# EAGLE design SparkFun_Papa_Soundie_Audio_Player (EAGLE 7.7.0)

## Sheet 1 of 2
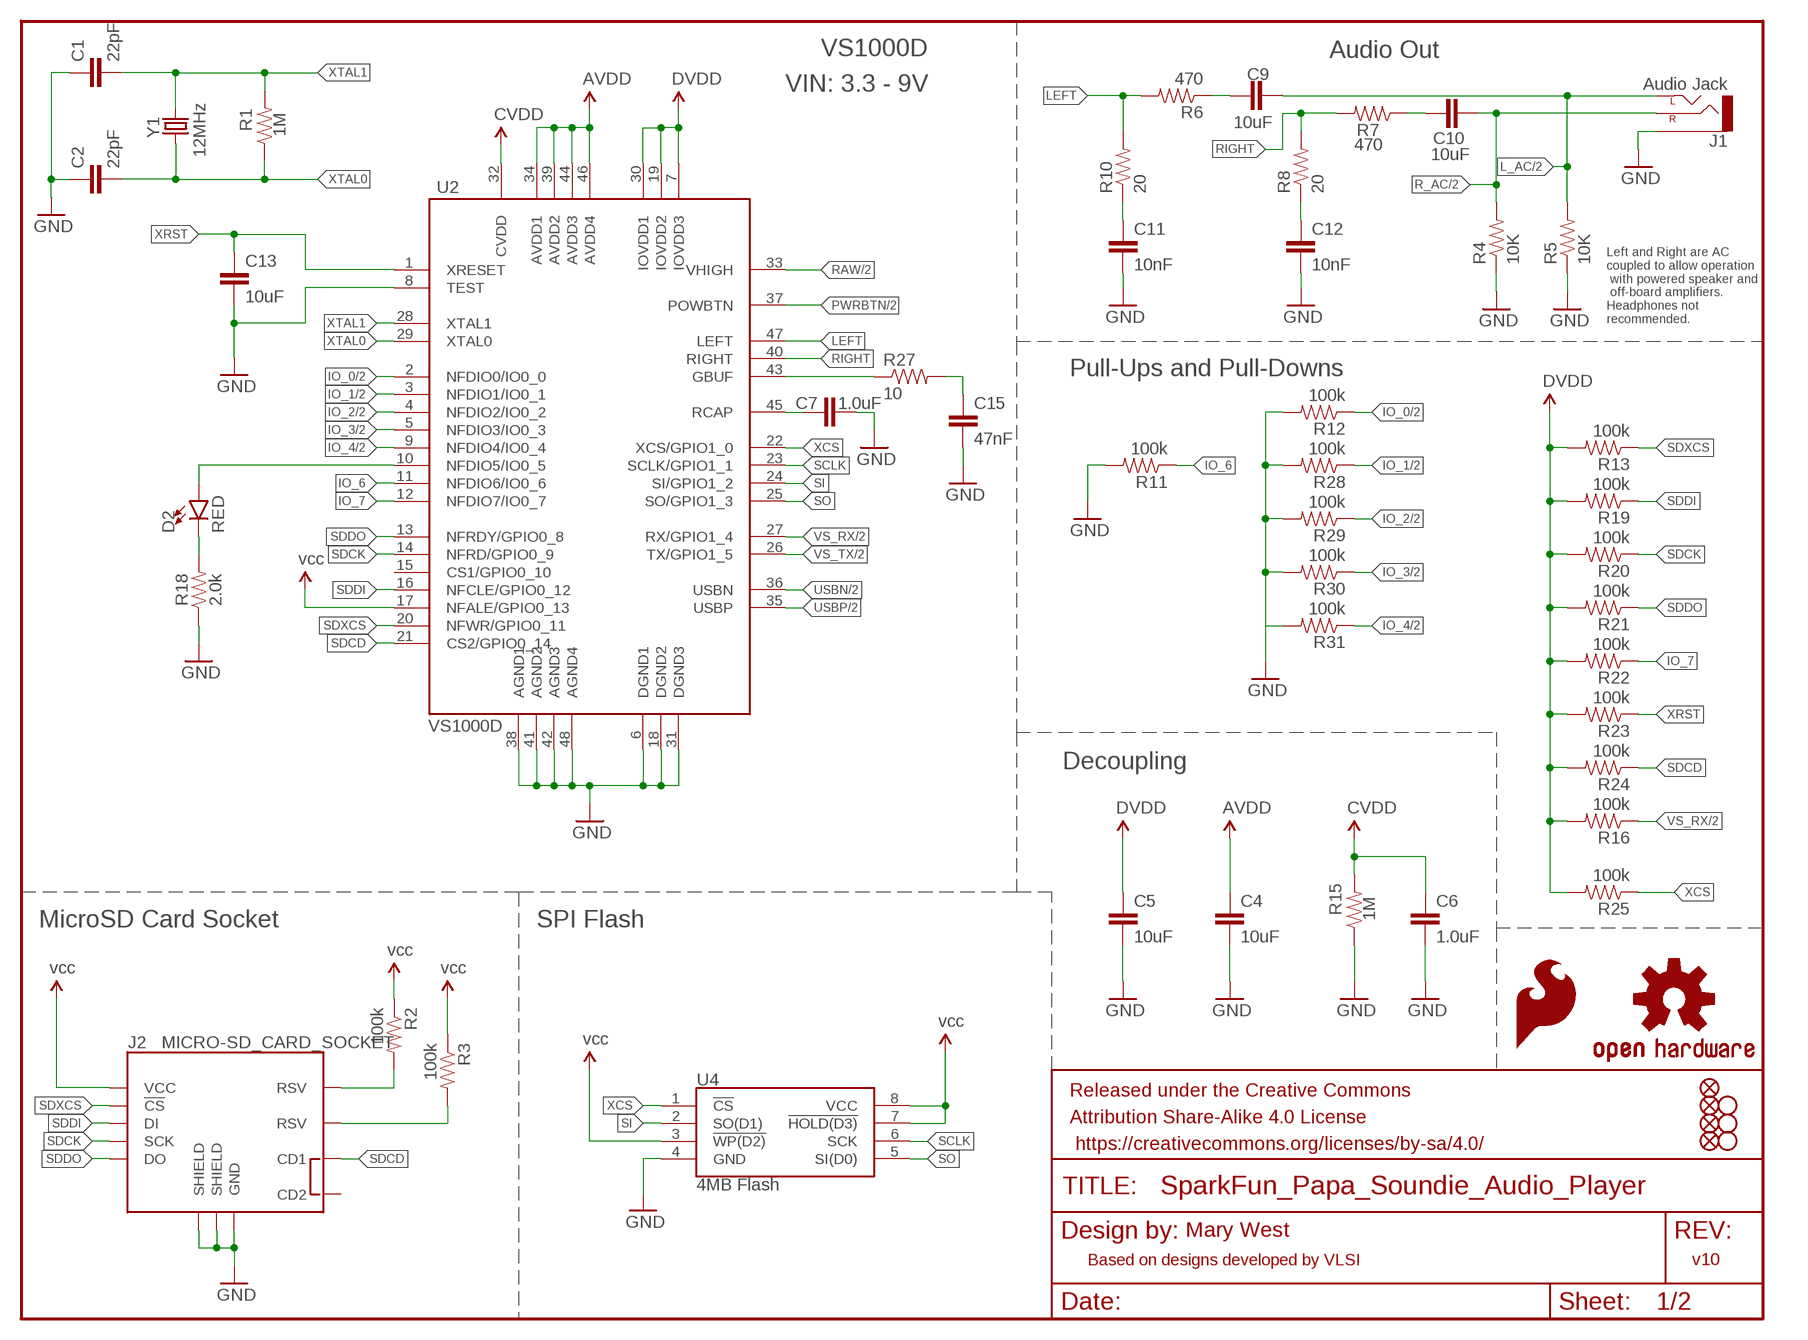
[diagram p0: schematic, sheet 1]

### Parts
C1  22pF  22PF-50V-5%(0603)  [0603-CAP]
C2  22pF  22PF-50V-5%(0603)  [0603-CAP]
C4  10uF  10UF-0603-6.3V-20%  [0603]
C5  10uF  10UF-0603-6.3V-20%  [0603]
C6  1.0uF  1.0UF-16V-10%(0603)  [0603-CAP]
C7  1.0uF  1.0UF-16V-10%(0603)  [0603-CAP]
C9  10uF  10UF-6.3V-20%(0603)  [0603-CAP]
C10  10uF  10UF-6.3V-20%(0603)  [0603-CAP]
C11  10nF  10NF/10000PF-50V-10%(0603)  [0603-CAP]
C12  10nF  10NF/10000PF-50V-10%(0603)  [0603-CAP]
C13  10uF  10UF-6.3V-20%(0603)  [0603-CAP]
C15  47nF  47NF(0.047UF/47000PF)-25V-5%(0603)SMD  [0603-CAP]
D2  RED  LED-RED0603  [LED-0603]
FD1  FIDUCIALUFIDUCIAL  [FIDUCIAL-MICRO]
FD2  FIDUCIALUFIDUCIAL  [FIDUCIAL-MICRO]
FD3  FIDUCIALUFIDUCIAL  [FIDUCIAL-MICRO]
FD4  FIDUCIALUFIDUCIAL  [FIDUCIAL-MICRO]
FRAME1  FRAME-LETTER  [CREATIVE_COMMONS]
H1  STAND-OFFTIGHT  [STAND-OFF-TIGHT]
H2  STAND-OFFTIGHT  [STAND-OFF-TIGHT]
H3  STAND-OFFTIGHT  [STAND-OFF-TIGHT]
J1  Audio Jack  AUDIO-JACKSMD2  [AUDIO-JACK-3.5MM-SMD]
J2  MICRO-SD_CARD_SOCKET  [MICRO-SD-SOCKET]
LOGO1  OSHW-LOGOL  [OSHW-LOGO-L]
LOGO2  SFE_LOGO_FLAME.2_INCH  [SFE_LOGO_FLAME_.2]
R1  1M  1MOHM-1/10W-1%(0603)  [0603-RES]
R2  100k  100KOHM-1/10W-1%(0603)  [0603-RES]
R3  100k  100KOHM-1/10W-1%(0603)  [0603-RES]
R4  10K  10KOHM-1/10W-1%(0603)0603  [0603-RES]
R5  10K  10KOHM-1/10W-1%(0603)0603  [0603-RES]
R6  470  470OHM1/10W1%(0603)  [0603-RES]
R7  470  470OHM1/10W1%(0603)  [0603-RES]
R8  20  20OHM1/10W1%(0603)SMD  [0603-RES]
R10  20  20OHM1/10W1%(0603)SMD  [0603-RES]
R11  100k  100KOHM-1/10W-1%(0603)  [0603-RES]
R12  100k  100KOHM-1/10W-1%(0603)  [0603-RES]
R13  100k  100KOHM-1/10W-1%(0603)  [0603-RES]
R15  1M  1MOHM-1/10W-1%(0603)  [0603-RES]
R16  100k  100KOHM-1/10W-1%(0603)  [0603-RES]
R18  2.0k  2.0KOHM-0603-1/10W-5%  [0603]
R19  100k  100KOHM-1/10W-1%(0603)  [0603-RES]
R20  100k  100KOHM-1/10W-1%(0603)  [0603-RES]
R21  100k  100KOHM-1/10W-1%(0603)  [0603-RES]
R22  100k  100KOHM-1/10W-1%(0603)  [0603-RES]
R23  100k  100KOHM-1/10W-1%(0603)  [0603-RES]
R24  100k  100KOHM-1/10W-1%(0603)  [0603-RES]
R25  100k  100KOHM-1/10W-1%(0603)  [0603-RES]
R27  10  10OHM-1/10W-5%0603SMD  [0603-RES]
R28  100k  100KOHM-1/10W-1%(0603)  [0603-RES]
R29  100k  100KOHM-1/10W-1%(0603)  [0603-RES]
R30  100k  100KOHM-1/10W-1%(0603)  [0603-RES]
R31  100k  100KOHM-1/10W-1%(0603)  [0603-RES]
U2  VS1000D  VS1000  [LQFP-48]
U4  4MB Flash  AT25SF041  [SO08]
Y1  12MHz  CRYSTALCRYSTAL-SMD-5X3-12MHZ  [CRYSTAL-SMD-5X3]

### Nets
AVDD: C4.1 U2.34(AVDD1) U2.39(AVDD2) U2.44(AVDD3) U2.46(AVDD4)
CVDD: C6.1 R15.2 U2.32(CVDD)
DVDD: C5.1 R13.2 R16.2 R19.2 R20.2 R21.2 R22.2 R23.2 R24.2 R25.2 U2.7(IOVDD3) U2.19(IOVDD2) U2.30(IOVDD1)
GBUF: R27.1 U2.43(GBUF)
GND: C1.1 C2.1 C4.2 C5.2 C6.2 C7.2 C11.2 C12.2 C13.2 C15.2 J1.SLEEVE J2.GND J2.GND1(SHIELD) J2.GND3(SHIELD) R4.1 R5.1 R11.2 R12.2 R15.1 R18.1 R28.2 R29.2 R30.2 R31.2 U2.6(DGND1) U2.8(TEST) U2.18(DGND2) U2.31(DGND3) U2.38(AGND1) U2.41(AGND2) U2.42(AGND3) U2.48(AGND4) U4.4(GND) ; also sheet 2
IO_0: R12.1 U2.2(NFDIO0/IO0_0) ; also sheet 2
IO_1: R28.1 U2.3(NFDIO1/IO0_1) ; also sheet 2
IO_2: R29.1 U2.4(NFDIO2/IO0_2) ; also sheet 2
IO_3: R30.1 U2.5(NFDIO3/IO0_3) ; also sheet 2
IO_4: R31.1 U2.9(NFDIO4/IO0_4) ; also sheet 2
IO_6: R11.1 U2.11(NFDIO6/IO0_6)
IO_7: R22.1 U2.12(NFDIO7/IO0_7)
L_AC: C9.2 J1.TIP(LEFT) R5.2 ; also sheet 2
LEFT: R6.2 R10.2 U2.47(LEFT)
N$2: C15.1 R27.2
N$3: C9.1 R6.1
N$6: C11.1 R10.1
N$7: C7.1 U2.45(RCAP)
N$15: J2.RSV1(RSV) R2.2
N$17: C10.1 R7.1
N$19: J2.RSV2(RSV) R3.2
N$20: C12.1 R8.1
N$34: D2.C R18.2
N$35: D2.A U2.10(NFDIO5/IO0_5)
PWRBTN: U2.37(POWBTN) ; also sheet 2
R_AC: C10.2 J1.RING(RIGHT) R4.2 ; also sheet 2
RAW: U2.33(VHIGH) ; also sheet 2
RIGHT: R7.2 R8.2 U2.40(RIGHT)
SCLK: U2.23(SCLK/GPIO1_1) U4.6(SCK)
SDCD: J2.CD1 R24.1 U2.21(CS2/GPIO0_14)
SDCK: J2.SCLK(SCK) R20.1 U2.14(NFRD/GPIO0_9)
SDDI: J2.DI R19.1 U2.16(NFCLE/GPIO0_12)
SDDO: J2.DO R21.1 U2.13(NFRDY/GPIO0_8)
SDXCS: J2.CS(!CS) R13.1 U2.20(NFWR/GPIO0_11)
SI: U2.24(SI/GPIO1_2) U4.2(SO(D1))
SO: U2.25(SO/GPIO1_3) U4.5(SI(D0))
USBN: U2.36(USBN) ; also sheet 2
USBP: U2.35(USBP) ; also sheet 2
VCC: J2.VCC R2.1 R3.1 U2.17(NFALE/GPIO0_13) U4.3(!WP(D2)) U4.7(!HOLD(D3)) U4.8(VCC) ; supply symbol labelled vcc ; also sheet 2
VS_RX: R16.1 U2.27(RX/GPIO1_4) ; also sheet 2
VS_TX: U2.26(TX/GPIO1_5) ; also sheet 2
XCS: R25.1 U2.22(XCS/GPIO1_0) U4.1(!CS)
XRST: C13.1 R23.1 U2.1(XRESET)
XTAL0: C2.2 R1.1 U2.29(XTAL0) Y1.1
XTAL1: C1.2 R1.2 U2.28(XTAL1) Y1.3
Unconnected: J2.CD2 U2.15(CS1/GPIO0_10)

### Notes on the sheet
- VS1000D | Audio Out
- VIN: 3.3 - 9V
- Left and Right are AC
  coupled to allow operation
   with powered speaker and
   off-board amplifiers.
  Headphones not 
  recommended.
- Pull-Ups and Pull-Downs
- Decoupling
- MicroSD Card Socket | SPI Flash
- Mary West
- Based on designs developed by VLSI | v10

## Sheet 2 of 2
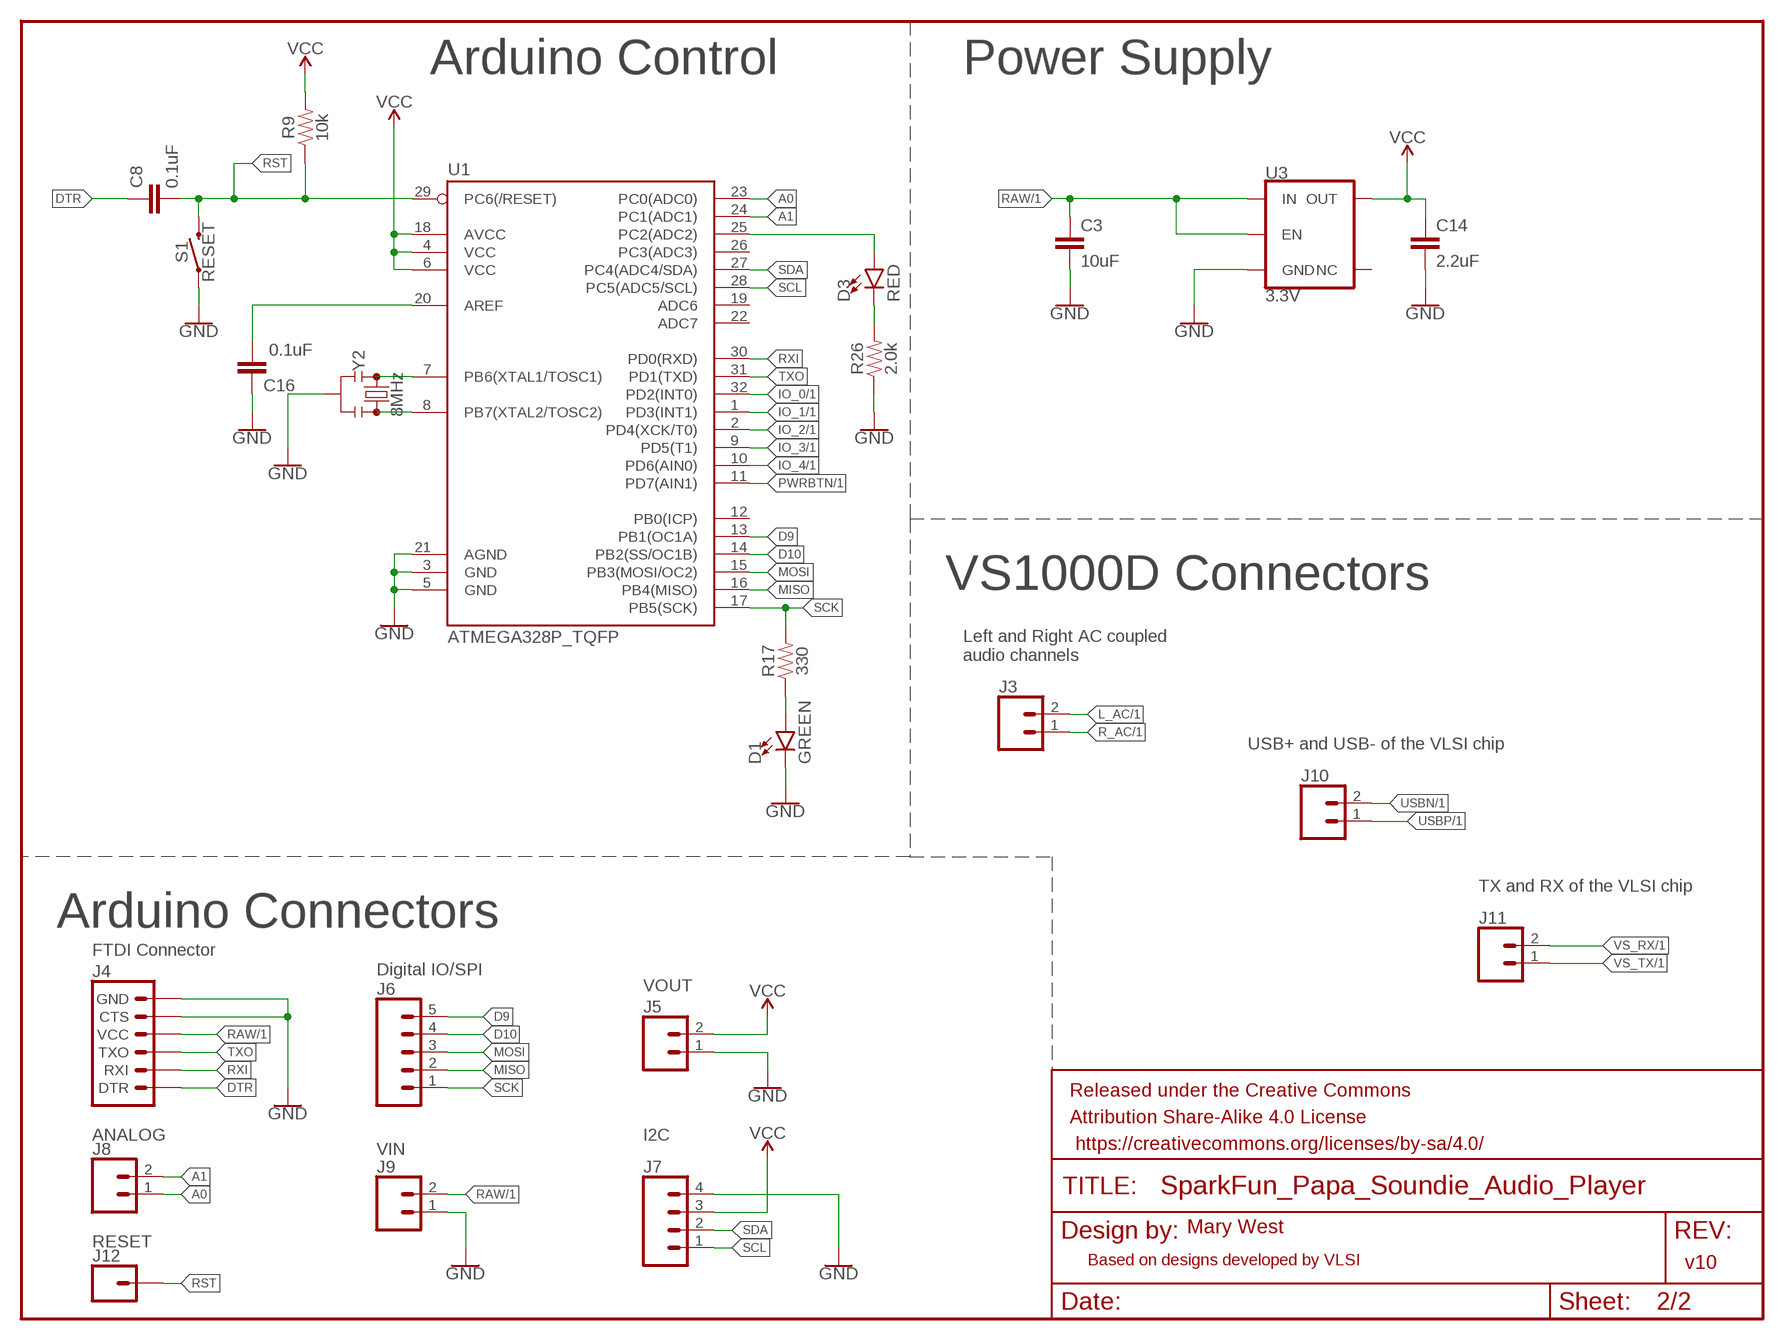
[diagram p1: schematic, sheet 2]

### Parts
C3  10uF  10UF-0603-6.3V-20%  [0603]
C8  0.1uF  0.1UF-0603-25V-(+80/-20%)  [0603]
C14  2.2uF  2.2UF-0603-10V-20%  [0603]
C16  0.1uF  0.1UF-0603-25V-(+80/-20%)  [0603]
D1  GREEN  LED-GREEN0603  [LED-0603]
D3  RED  LED-RED0603  [LED-0603]
FRAME2  FRAME-LETTER  [CREATIVE_COMMONS]
J3  CONN_02  [1X02]
J4  6_PIN_SERIAL_TARGETSILK  [6_PIN_SERIAL_TARGET_SIDE_W_SILK]
J5  CONN_02  [1X02]
J6  CONN_05  [1X05]
J7  CONN_04  [1X04]
J8  CONN_02  [1X02]
J9  CONN_02  [1X02]
J10  CONN_02  [1X02]
J11  CONN_02  [1X02]
J12  CONN_01  [1X01]
R9  10k  10KOHM-0603-1/10W-1%  [0603]
R17  330  330OHM-0603-1/10W-1%  [0603]
R26  2.0k  2.0KOHM-0603-1/10W-5%  [0603]
S1  RESET  MOMENTARY-SWITCH-SPST-SMD-5.2MM  [TACTILE_SWITCH_SMD_5.2MM]
U1  ATMEGA328P_TQFP  [TQFP32-08]
U3  3.3V  V_REG_AP2112K-3.3V  [SOT23-5]
Y2  8MHz  RESONATOR-8MHZSMD_3.2X1.3  [RESONATOR-SMD-3.2X1.3]

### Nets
A0: J8.1 U1.23(PC0(ADC0))
A1: J8.2 U1.24(PC1(ADC1))
D9: J6.5 U1.13(PB1(OC1A))
D10: J6.4 U1.14(PB2(SS/OC1B))
DTR: C8.1 J4.P$1(DTR)
GND: C3.2 C14.2 C16.1 D1.C J4.P$5(CTS) J4.P$6(GND) J5.1 J7.4 J9.1 R26.1 S1.1 U1.3(GND) U1.5(GND) U1.21(AGND) U3.2(GND) Y2.2 ; also sheet 1
IO_0: U1.32(PD2(INT0)) ; also sheet 1
IO_1: U1.1(PD3(INT1)) ; also sheet 1
IO_2: U1.2(PD4(XCK/T0)) ; also sheet 1
IO_3: U1.9(PD5(T1)) ; also sheet 1
IO_4: U1.10(PD6(AIN0)) ; also sheet 1
L_AC: J3.2 ; also sheet 1
MISO: J6.2 U1.16(PB4(MISO))
MOSI: J6.3 U1.15(PB3(MOSI/OC2))
N$8: U1.7(PB6(XTAL1/TOSC1)) Y2.1
N$16: U1.8(PB7(XTAL2/TOSC2)) Y2.3
N$31: D3.A U1.25(PC2(ADC2))
N$36: D3.C R26.2
N$39: C16.2 U1.20(AREF)
N$42: D1.A R17.1
PWRBTN: U1.11(PD7(AIN1)) ; also sheet 1
R_AC: J3.1 ; also sheet 1
RAW: C3.1 J4.P$4(VCC) J9.2 U3.1(IN) U3.3(EN) ; also sheet 1
RST: C8.2 J12.1 R9.1 S1.3 U1.29(PC6(/RESET))
RXI: J4.P$3(RXI) U1.30(PD0(RXD))
SCK: J6.1 R17.2 U1.17(PB5(SCK))
SCL: J7.1 U1.28(PC5(ADC5/SCL))
SDA: J7.2 U1.27(PC4(ADC4/SDA))
TXO: J4.P$2(TXO) U1.31(PD1(TXD))
USBN: J10.2 ; also sheet 1
USBP: J10.1 ; also sheet 1
VCC: C14.1 J5.2 J7.3 R9.2 U1.4(VCC) U1.6(VCC) U1.18(AVCC) U3.5(OUT) ; also sheet 1
VS_RX: J11.2 ; also sheet 1
VS_TX: J11.1 ; also sheet 1
Unconnected: U1.12(PB0(ICP)) U1.19(ADC6) U1.22(ADC7) U1.26(PC3(ADC3)) U3.4(NC)

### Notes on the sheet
- Arduino Control | Power Supply
- VS1000D Connectors
- Left and Right AC coupled 
  audio channels
- USB+ and USB- of the VLSI chip
- TX and RX of the VLSI chip
- Arduino Connectors
- FTDI Connector
- Digital IO/SPI
- VOUT
- ANALOG | I2C
- VIN
- Mary West
- RESET
- Based on designs developed by VLSI | v10

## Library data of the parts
C1 C2 = SparkFun-Capacitors:22PF-50V-5%(0603): CAP-07876; PROD_ID: CAP-07876
C3-C5 = SparkFun-Capacitors:10UF: 10.0µF ceramic capacitors; PROD_ID: CAP-11015
C6 C7 = SparkFun-Capacitors:1.0UF-16V-10%(0603): CAP-00868; PROD_ID: CAP-00868
C8 C16 = SparkFun-Capacitors:0.1UF: 0.1µF ceramic capacitors; PROD_ID: CAP-00810
C9 C10 C13 = SparkFun-Capacitors:10UF-6.3V-20%(0603): CAP-11015; PROD_ID: CAP-11015
C11 C12 = SparkFun-Capacitors:10NF/10000PF-50V-10%(0603): CAP-00867; PROD_ID: CAP-00867
C14 = SparkFun-Capacitors:2.2UF: 2.2µF ceramic capacitors; PROD_ID: CAP-07888
C15 = SparkFun-Capacitors:47NF(0.047UF/47000PF)-25V-5%(0603): CAP-08605; PROD_ID: CAP-08605
D1 = SparkFun-LED:LED-GREEN: Green SMD LED; PROD_ID: DIO-00821
D2 D3 = SparkFun-LED:LED-RED: Red SMD LED; PROD_ID: DIO-00819
FD1-FD4 = SparkFun-Aesthetics:FIDUCIAL: Fiducial Alignment Points
FRAME1 FRAME2 = SparkFun-Aesthetics:FRAME-LETTER: Schematic Frame - Letter
H1-H3 = SparkFun-Electromechanical:STAND-OFF: #4 Stand Off
J1 = SparkFun-Connectors:AUDIO-JACK: 3.5mm Audio Jack Simple 3.5mm common PCB mount audio jack. Variant PTH is our storefront SKU PRT-08032; PROD_ID: CONN-10353
J2 = SparkFun-Connectors:MICRO-SD_CARD_SOCKET: microSD Socket for Transflash Push-push type µSD socket. tDoc lines correctly indicate media card edge positions when inserting (unlocked, locked, depressed). NOTE: CD1 and CD2 are connected internally, and the default detect state of the socket is detect pin to ground. SparkFun Products: WAV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; PROD_ID: CONN-07820; SF_ID: PRT-00127
J3 J5 J8-J11 = SparkFun-Connectors:CONN_02: Multi connection point. Often used as Generic Header-pin footprint for 0.1 inch spaced/style header connections
J4 = SparkFun-Connectors:6_PIN_SERIAL_TARGET: 6-pin header connection for use with the "FTDI BASIC" pinout - TARGET SIDE. Also known as "Arduino Serial Program Header". It is used to mate with our FTDI Basic serial programmers using the Arduino IDE. Note, this device has "TARGET" in the name. It is intended to be used on a design that contains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
J6 = SparkFun-Connectors:CONN_05: Multi connection point. Often used as Generic Header-pin footprint for 0.1 inch spaced/style header connections On any of the 0.1 inch spaced packages, you can populate with these: Break Away Headers - Straight (PRT-00116) Break Away Male Headers - Right Angle (PRT-00553) Female Headers (PRT-00115)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
J7 = SparkFun-Connectors:CONN_04: Multi connection point. Often used as Generic Header-pin footprint for 0.1 inch spaced/style header connections On any of the 0.1 inch spaced packages, you can populate with these: Break Away Headers - Straight (PRT-00116) Break Away Male Headers - Right Angle (PRT-00553) Female Headers (PRT-00115)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; PROD_ID: CONN-09696
J12 = SparkFun-Connectors:CONN_01: Single connection point. Often used as Generic Header-pin footprint for 0.1 inch spaced/style header connections
LOGO1 = SparkFun-Aesthetics:OSHW-LOGO: Open-Source Hardware (OSHW) Logo
LOGO2 = SparkFun-Aesthetics:SFE_LOGO_FLAME: SparkFun Flame Logo
R1 R15 = SparkFun-Resistors:1MOHM-1/10W-1%(0603): RES-07868; PROD_ID: RES-07868
R2 R3 R11-R13 R16 R19-R25 R28-R31 = SparkFun-Resistors:100KOHM-1/10W-1%(0603): RES-07828; PROD_ID: RES-07828
R4 R5 = SparkFun-Resistors:10KOHM-1/10W-1%(0603): RES-00824; PROD_ID: RES-00824
R6 R7 = SparkFun-Resistors:470OHM1/10W1%(0603): RES-07869; PROD_ID: RES-07869
R8 R10 = SparkFun-Resistors:20OHM1/10W1%(0603): RES-07862; PROD_ID: RES-07862
R9 = SparkFun-Resistors:10KOHM: 10kΩ resistor; PROD_ID: RES-00824
R17 = SparkFun-Resistors:330OHM: 330Ω resistor; PROD_ID: RES-00818
R18 R26 = SparkFun-Resistors:2.0KOHM: 2kΩ resistor; PROD_ID: RES-08296
R27 = SparkFun-Resistors:10OHM-1/10W-5%0603: RES-09834; PROD_ID: RES-09834
S1 = SparkFun-Switches:MOMENTARY-SWITCH-SPST: Momentary Switch (Pushbutton) - SPST; PROD_ID: SWCH-08247; SF_SKU: COM-08720
U1 = SparkFun-IC-Microcontroller:ATMEGA328P_TQFP: Popular 328P in QFP Storefront component: ATmega328 - TQFP (COM-13448) Datasheet SparkFun Products SparkFun RedBoard - Programmed with Arduino (DEV-12757) Arduino Pro Mini 328 - 5V/16MHz (DEV-11113) Arduino Pro Mini 328 - 3.3V/8MHz (DEV-11114) SparkFun OpenLog (DEV-13712) SparkFun MicroView - OLED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; PROD_ID: IC-09069
U2 = SparkFun-IC-Conversion:VS1000: VS1000D Ogg Vorbis Player IC with USB and NAND FLASH Interface 12 MHz LQFP-48 Datasheet SparkFun Products Storefront component: Ogg Vorbis Codec IC - VS1000D (COM-08300); PROD_ID: LPA-12743
U3 = SparkFun-IC-Power:V_REG_AP2112: AP2112 - 600mA CMOS LDO Regulator w/ Enable The AP2112 is CMOS process low dropout linear regulator with enable function, the regulator delivers a guaranteed 600mA (min.) continuous load current. Features Output Voltage Accuracy: ±1.5% Output Current: 600mA (Min.) Foldback Short Current Protection: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; PROD_ID: VREG-12457
U4 = SparkFun-IC-Memory:AT25SF041: AT25SF041 4Mb Serial Flash Memory 104MHz, SPI, 8-SOIC Datasheet SparkFun Products: SparkFun ESP8266 Thing SparkFun ESP8266 Thing - Dev Board; PROD_ID: IC-12455
Y1 = SparkFun-FreqCtrl:CRYSTAL: Various standard crystals. Proven footprints.; PROD_ID: XTAL-08297
Y2 = SparkFun-Clocks:RESONATOR-8MHZ: 8MHz Resonator Digikey Example Frequency: 8MHz Frequency Stability: &plusmn;0.2% Frequency Tolerance: &plusmn;0.5% Capacitance: 33pF SparkFun Products Arduino Pro Mini 328- 3.3V/8MHz SparkFun Digital Sandbox; PROD_ID: XTAL-08895

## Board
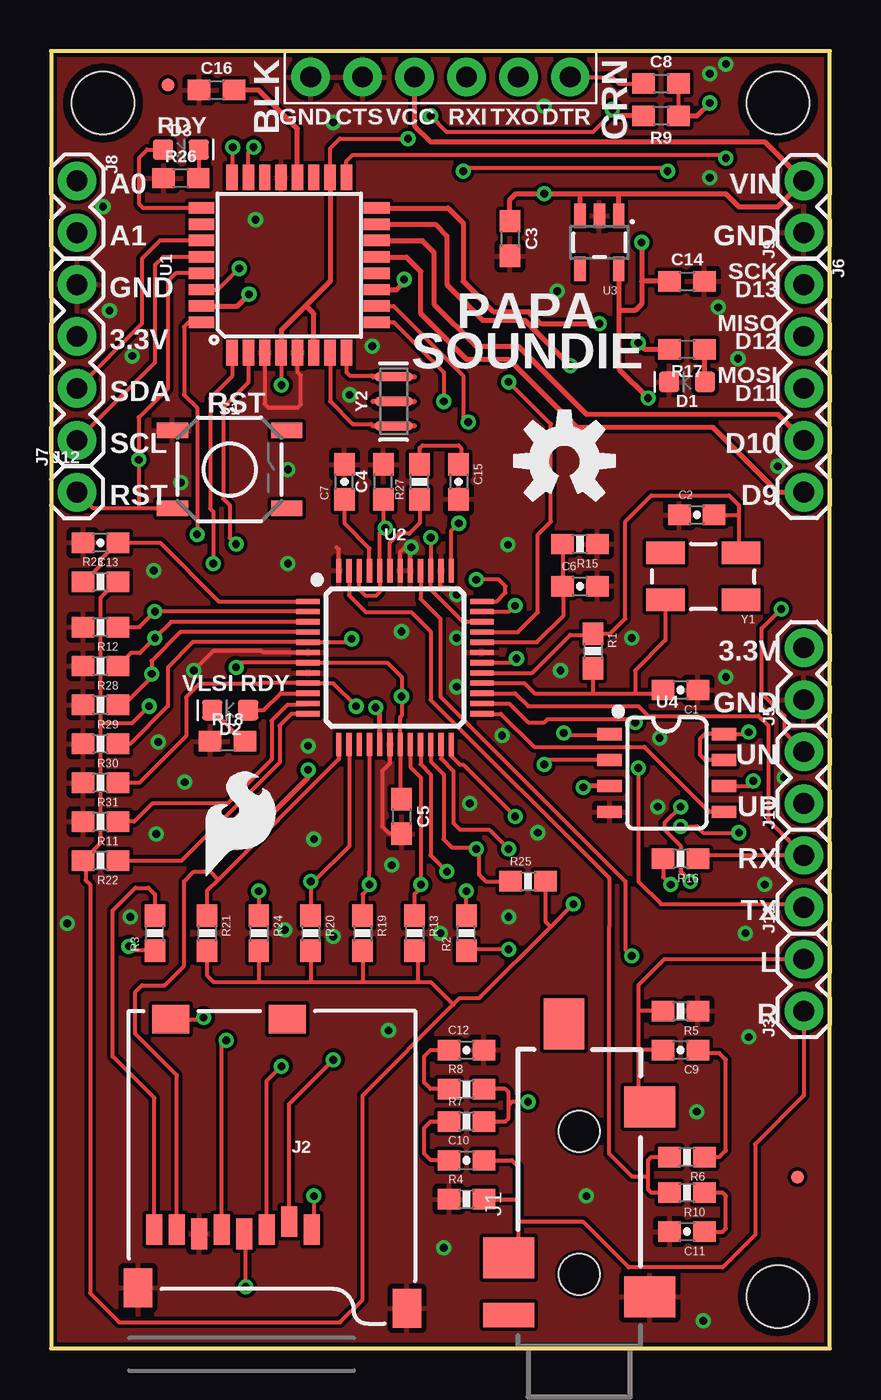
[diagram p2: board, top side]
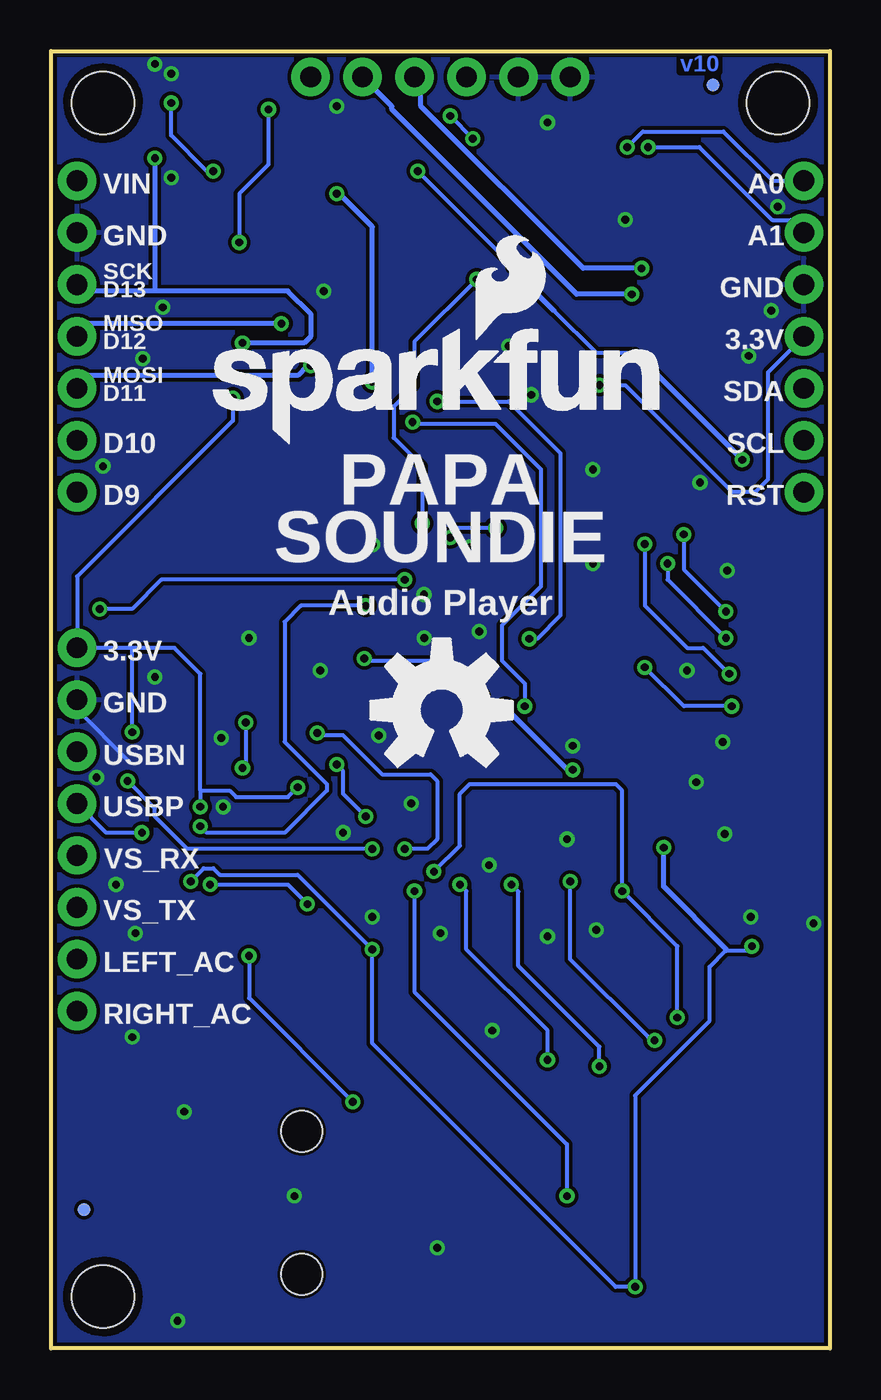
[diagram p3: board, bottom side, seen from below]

Size 38.1 x 63.5 mm. Coordinates in mm from the lower left corner, seen from the top.
Outline: 38.1,63.5 0,63.5 0,0 38.1,0 38.1,63.5
Copper layers (1*16): Top 0.035mm / dielectric 1.5mm / Bottom 0.035mm
Design rules "SparkFun-2-layer-TIGHT": minimum track width 7mil, minimum drill 15mil, track to track 7mil, track to pad 7mil, pad to pad 7mil, via to via 7mil, smd to smd 7mil, copper to edge 7mil, drill to drill 7mil, minimum pad ring 7mil, minimum via ring 7mil, stop-mask expansion 4mil, vias tented up to drill 25mil, thermal gap 10mil

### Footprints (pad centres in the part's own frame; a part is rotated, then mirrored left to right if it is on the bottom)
0603-CAP = smd 1.1 x 1: 1 -0.85,0; 2 0.85,0
0603 = smd 1.1 x 1: 1 -0.85,0; 2 0.85,0
LED-0603 = smd 1 x 1: A -0.877,0; C 0.877,0
FIDUCIAL-MICRO = smd 0.635 x 0.635: 1 0,0
STAND-OFF-TIGHT = hole 3.048: 0,0
AUDIO-JACK-3.5MM-SMD = smd 2 x 2.5: RING 4.3,3.45; SLEEVE 2.4,-3.45; TIP 11.7,-3.45 | smd 1.2 x 2.5: RSH 1.5,3.45 | smd 2.5 x 2: TSH 15.75,0.75 | hole 2: 3.5,0; 10.5,0
MICRO-SD-SOCKET = smd 1.8 x 1.4: CD1 -2.05,0.4; CD2 -7.75,0.4 | smd 0.8 x 1.5: CS -7.84,10.3; DI -6.74,10.7; DO -2.34,10.7; GND -3.44,10.9; RSV1 -8.94,10.7; RSV2 -1.24,10.7; SCLK -4.54,10.7; VCC -5.64,10.9 | smd 1.4 x 1.9: GND1 -13.6,14.55; GND3 -0.45,13.55
1X02 = drill 1.016 pad 1.88: 1 0,0; 2 2.54,0
6_PIN_SERIAL_TARGET_SIDE_W_SILK = drill 1.016 pad 1.88: P$1 -6.35,0; P$2 -3.81,0; P$3 -1.27,0; P$4 1.27,0; P$5 3.81,0; P$6 6.35,0
1X05 = drill 1.016 pad 1.88: 1 0,0; 2 2.54,0; 3 5.08,0; 4 7.62,0; 5 10.16,0
1X04 = drill 1.016 pad 1.88: 1 0,0; 2 2.54,0; 3 5.08,0; 4 7.62,0
1X01 = drill 1.016 pad 1.88: 1 0,0
0603-RES = smd 1.1 x 1: 1 -0.85,0; 2 0.85,0
TACTILE_SWITCH_SMD_5.2MM = smd 1.524 x 0.762: 1 -2.794,1.905; 2 2.794,1.905; 3 -2.794,-1.905; 4 2.794,-1.905
TQFP32-08 = smd 1.27 x 0.559: 1 -4.293,2.8; 2 -4.293,2; 3 -4.293,1.2; 4 -4.293,0.4; 5 -4.293,-0.4; 6 -4.293,-1.2; 7 -4.293,-2; 8 -4.293,-2.8; 17 4.293,-2.8; 18 4.293,-2; 19 4.293,-1.2; 20 4.293,-0.4; 21 4.293,0.4; 22 4.293,1.2; 23 4.293,2; 24 4.293,2.8 | smd 0.559 x 1.27: 9 -2.8,-4.293; 10 -2,-4.293; 11 -1.2,-4.293; 12 -0.4,-4.293; 13 0.4,-4.293; 14 1.2,-4.293; 15 2,-4.293; 16 2.8,-4.293; 25 2.8,4.293; 26 2,4.293; 27 1.2,4.293; 28 0.4,4.293; 29 -0.4,4.293; 30 -1.2,4.293; 31 -2,4.293; 32 -2.8,4.293
LQFP-48 = smd 0.254 x 1.143: 1 -2.75,-4.25; 2 -2.25,-4.25; 3 -1.75,-4.25; 4 -1.25,-4.25; 5 -0.75,-4.25; 6 -0.25,-4.25; 7 0.25,-4.25; 8 0.75,-4.25; 9 1.25,-4.25; 10 1.75,-4.25; 11 2.25,-4.25; 12 2.75,-4.25; 25 2.75,4.25; 26 2.25,4.25; 27 1.75,4.25; 28 1.25,4.25; 29 0.75,4.25; 30 0.25,4.25; 31 -0.25,4.25; 32 -0.75,4.25; 33 -1.25,4.25; 34 -1.75,4.25; 35 -2.25,4.25; 36 -2.75,4.25 | smd 1.143 x 0.254: 13 4.25,-2.75; 14 4.25,-2.25; 15 4.25,-1.75; 16 4.25,-1.25; 17 4.25,-0.75; 18 4.25,-0.25; 19 4.25,0.25; 20 4.25,0.75; 21 4.25,1.25; 22 4.25,1.75; 23 4.25,2.25; 24 4.25,2.75; 37 -4.25,2.75; 38 -4.25,2.25; 39 -4.25,1.75; 40 -4.25,1.25; 41 -4.25,0.75; 42 -4.25,0.25; 43 -4.25,-0.25; 44 -4.25,-0.75; 45 -4.25,-1.25; 46 -4.25,-1.75; 47 -4.25,-2.25; 48 -4.25,-2.75
SOT23-5 = smd 0.55 x 1.2: 1 -0.95,-1.3; 2 0,-1.3; 3 0.95,-1.3; 4 0.95,1.3; 5 -0.95,1.3
SO08 = smd 0.6 x 1.2: 1 -1.905,-2.8; 2 -0.635,-2.8; 3 0.635,-2.8; 4 1.905,-2.8; 5 1.905,2.8; 6 0.635,2.8; 7 -0.635,2.8; 8 -1.905,2.8
CRYSTAL-SMD-5X3 = smd 1.9 x 1.1: 1 -1.85,-1.15; 2 1.85,-1.15; 3 1.85,1.15; 4 -1.85,1.15
RESONATOR-SMD-3.2X1.3 = smd 0.45 x 1.905: 1 -1.2,0; 2 0,0; 3 1.2,0

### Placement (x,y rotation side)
C1  30.8,32.23 180 top
C2  31.59,40.8 0 top
C3  22.45,54.32 270 top
C4  16.26,42.42 90 top
C5  17.14,26.04 270 top
C6  25.88,37.31 0 top
C7  14.35,42.42 90 top
C8  29.84,61.91 0 top
C9  30.8,14.61 180 top
C10  20.32,9.21 0 top
C11  31.11,5.71 180 top
C12  20.32,14.61 0 top
C13  2.41,39.43 180 top
C14  31.11,52.23 0 top
C15  19.94,42.42 270 top
C16  8.1,61.59 0 top
D1  31.11,47.31 180 top
D2  8.76,31.24 180 top
D3  6.35,58.67 0 top
FD1  5.71,61.85 90 top
FD2  36.51,8.38 90 top
FD3  5.71,61.85 180 bottom
FD4  36.48,6.79 180 bottom
FRAME1  not placed on the board
FRAME2  not placed on the board
FRAME3  FRAME-LETTER  [CREATIVE_COMMONS]  not placed on the board
H1  35.56,60.96 90 top
H2  2.54,60.96 180 top
H3  35.56,2.54 0 top
J1  25.84,0.13 90 top
J2  3.81,16.51 180 top
J3  36.83,16.51 90 top
J4  19.05,62.23 180 top
J5  36.83,31.75 90 top
J6  36.83,52.07 270 top
J7  1.27,44.45 90 top
J8  1.27,57.15 270 top
J9  36.83,54.61 90 top
J10  36.83,26.67 90 top
J11  36.83,21.59 90 top
J12  1.27,41.91 0 top
LOGO1  18.99,31.24 0 bottom
LOGO2  7.24,22.86 0 top
LOGO3  OSHW-LOGOL  [OSHW-LOGO-M]  25.11,43.43 0 top
LOGO6  SFE_LOGO_NAME_FLAME.1_INCH  [SFE_LOGO_NAME_FLAME_.2]  30.87,44.2 0 bottom
R1  26.51,34.13 270 top
R2  20.32,20.32 90 top
R3  5.08,20.32 90 top
R4  20.32,7.3 0 top
R5  30.8,16.51 180 top
R6  31.11,9.37 180 top
R7  20.32,11.11 0 top
R8  20.32,12.7 0 top
R9  29.84,60.33 180 top
R10  31.11,7.62 180 top
R11  2.41,25.78 180 top
R12  2.41,35.31 180 top
R13  17.78,20.32 270 top
R15  25.88,39.37 180 top
R16  30.8,23.97 180 top
R17  31.11,48.9 180 top
R18  8.64,29.72 0 top
R19  15.24,20.32 270 top
R20  12.7,20.32 270 top
R21  7.62,20.32 270 top
R22  2.41,23.88 180 top
R23  2.41,37.53 0 top
R24  10.16,20.32 270 top
R25  23.34,22.86 0 top
R26  6.35,57.28 0 top
R27  18.03,42.42 90 top
R28  2.41,33.4 180 top
R29  2.41,31.5 180 top
R30  2.41,29.59 180 top
R31  2.41,27.69 180 top
S1  8.73,43.02 0 top
U1  11.65,53.02 90 top
U2  16.83,33.81 270 top
U3  26.83,54.13 180 top
U4  30.13,28.16 270 top
Y1  31.91,37.78 180 top
Y2  16.76,46.35 90 top

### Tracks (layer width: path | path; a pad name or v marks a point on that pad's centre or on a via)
A0  (via drill 0.38)
  Top 0.203: U1.23 9.65,58.55 v9.91,58.8 10.03,58.93
  Bottom 0.203: v9.91,58.8 9.14,59.56 5.21,59.56 2.79,57.15 J8.1
A1  (via drill 0.38)
  Top 0.203: U1.24 8.89,57.35 v8.89,58.8
  Bottom 0.203: J8.2 1.89,55.23 2.81,55.23 6.38,58.8 v8.89,58.8
AVDD  (via drill 0.38)
  Top 0.203: U2.34 20.16,35.56 18.57,37.15 U2.39 v18.57,39.69 | U2.46 15.08,37.15 15.4,36.83 15.88,36.83 16.08,37.03 U2.44 16.08,39.89 v16.35,40.16 | 16.29,40.23 v16.35,40.16 | C4.1 16.26,40.26 v16.35,40.16
  Bottom 0.203: v16.35,40.16 18.26,40.16 18.57,39.85 v18.57,39.69
CVDD
  Top 0.203: U2.32 23.77,34.56 25.08,35.88 25.08,37.25 C6.1 R15.2
D9
  Top 0.254: U1.13 17.38,53.42 18.1,52.7 18.1,50.64 20.32,48.42 22.38,48.42 25.72,45.09 32.38,45.09 35.56,41.91 J6.5
D10
  Top 0.254: U1.14 18.17,54.22 18.73,53.66 18.73,51.12 20.8,49.05 22.86,49.05 26.19,45.72 35.56,45.72 J6.4
DTR
  Top 0.203: J4.P$1 27.46,62.23 27.78,61.91 C8.1
DVDD  (via drill 0.38)
  Top 0.203: C5.1 17.08,26.95 U2.19 17.08,30.89 17.14,30.96 v17.14,31.91 17.14,32.86 16.44,33.56 U2.7 9.28,33.56 v9.05,33.34 | R21.2 7.62,18.26 7.94,17.94 10.16,17.94 | 10.16,17.94 12.7,17.94 | 12.7,17.94 15.24,17.94 | 15.24,17.94 17.94,17.94 | 17.94,17.94 18.57,17.94 19.68,16.83 | R13.2 17.94,19.31 17.94,17.94 | R19.2 15.24,17.94 | R24.2 10.16,17.94 | R20.2 12.7,17.94 | R23.2 3.21,37.53 2.41,36.73 2.41,30.61 | 2.41,30.61 2.41,24.73 R22.2 1.69,23.75 1.69,22.92 1.91,22.7 1.91,2.7 3.33,1.27 14.13,1.27 15.24,2.38 15.24,12.38 19.68,16.83 | 19.68,16.83 20,17.14 20.95,17.14 24.45,20.64 | 24.45,20.64 v25.56,21.75 | R16.2 29.95,23.07 v30.32,22.7 | U2.30 22.56,33.56 v22.77,33.77 | R25.2 24.19,20.9 24.45,20.64 | 2.41,30.61 3.97,30.61 v4.79,31.43
  Bottom 0.203: v17.14,31.91 18.89,33.66 22.65,33.66 v22.77,33.77 | v30.32,22.7 26.51,22.7 v25.56,21.75 | v4.79,31.43 7.14,31.43 v9.05,33.34
GBUF
  Top 0.203: U2.43 16.58,39.44 17.02,39.88 17.53,39.88 18.03,40.39 R27.1
GND  (via drill 0.38)
  Top 0.203: U2.6 10.39,34.06 10.32,34.13 7.94,34.13 v6.99,33.18 | U2.18 16.58,28.64 16.19,28.26 16.19,25.56 16.51,25.24 17.09,25.24 C5.2 | U1.3 10.45,46.22 10.64,46.04 12.06,46.04 12.22,46.2 12.22,47.62 12.06,47.78 12.06,48.72 U1.5 | U2.48 14.08,39.1 13.97,39.21 | U2.41 17.58,39.1 17.46,39.21 17.3,39.21 17.08,38.98 U2.42 | v19.85,36.9 19.54,37.21 19.05,37.21 19.05,38.04 U2.38
  Bottom 0.203: J5.1 36.83,31.27 34.29,28.73
  other vias: 24.92,33.18 6.35,42.39 11.59,43.02 11.59,38.42 24.13,60.8 32.23,62.39 33.02,62.87 2.54,55.88 3.97,48.58 5.02,38.07 24.77,51.75 32.64,50.96 33.61,48.45 5.24,29.69 12.86,24.92 31.59,11.59 33.97,20.32 29.69,26.51 11.43,20.48 13.81,20.16 17.62,39.21 19.84,34.77 19.84,32.38 17.14,35.08 6.54,27.72 33.02,32.86 29.77,29.89 20.48,26.67 23.81,25.24 22.38,21.11 34.92,22.7 32.23,57.31 16.67,23.65 35.88,27.94 22.07,30 16.51,15.56 19.21,4.92 26.19,7.46 34.13,15.24 31.91,1.36 14.61,46.67 15.72,49.05 10,55.24 13.81,60.01 2.86,50.8 28.42,34.77 22.35,39.34 0.79,20.8 19.05,20.32 35.56,43.18 5.14,25.18 12.57,29.5 3.87,21.11
  pour Bottom: 38.1,0 0,0 0,63.5 38.1,63.5
  pour Top: 38.1,0 0,0 0,63.5 38.1,63.5
IO_0  (via drill 0.38)
  Top 0.203: U2.2 v5.08,36.06 4.32,35.31 R12.1 | U1.32 6.72,50.22 6.51,50.01 6.51,46.67 7.14,46.04 v7.14,39.85
  Bottom 0.203: v7.14,39.85 7.14,38.13 v5.08,36.06
IO_1  (via drill 0.38)
  Top 0.203: U2.3 5.88,35.56 v5.08,34.77 4.35,34.04 3.9,34.04 R28.1 | U1.1 8.85,47.59 7.78,46.51 7.78,41.12 7.94,40.96 v7.94,38.42
  Bottom 0.203: v7.94,38.42 7.94,37.62 v5.08,34.77
IO_2  (via drill 0.38)
  Top 0.203: U2.4 6.33,35.06 4.92,33.66 v4.92,33.02 4.92,32.86 3.56,31.5 R29.1 | U1.2 9.65,47.28 8.41,46.04 8.41,41.59 8.73,41.27 8.73,39.69 v9.05,39.37
  Bottom 0.203: v9.05,39.37 9.05,36.35 6.99,34.29 6.19,34.29 v4.92,33.02
IO_3  (via drill 0.38)
  Top 0.203: U1.9 16.77,50.22 19.21,47.78 v19.21,46.35 | R30.1 3.87,29.59 5.71,31.43 5.71,33.34 6.94,34.56 U2.5 14.53,34.56 v14.7,34.73
  Bottom 0.203: v19.21,46.35 15.72,46.35 13.18,43.81 13.18,35.88 14.32,34.73 v14.7,34.73
IO_4  (via drill 0.38)
  Top 0.203: U1.10 16.76,51.02 20.16,47.62 20.16,45.59 v20.41,45.34 | v14.92,31.43 13.79,32.56 U2.9 10.21,32.56 10.16,32.51 7.24,32.51 6.6,31.88 6.6,29.97 4.32,27.69 R31.1 3.39,27.81
  Bottom 0.203: v14.92,31.43 14.92,32.54 16.03,33.66 16.03,35.4 14.13,37.31 14.13,43.02 16.35,45.24 20.32,45.24 v20.41,45.34
IO_6
  Top 0.203: U2.11 12.51,31.5 11.56,31.5 10.79,30.73 10.79,28.83 8.64,26.67 4.95,26.67 4.06,25.78 R11.1
IO_7
  Top 0.203: U2.12 11.76,31.06 11.18,30.48 11.18,28.67 7.32,24.81 7.27,24.77 6.38,23.88 R22.1
L_AC
  Top 0.203: 28.73,14.61 28.73,12.39 J1.TIP | C9.2 28.73,14.61 | J3.2 30,19.05 28.73,17.78 28.73,16.51 | 28.73,16.51 28.73,14.61 | R5.2 28.73,16.51
LEFT
  Top 0.203: R10.2 29.37,7.62 29.21,7.78 29.21,8.41 | 29.21,8.41 29.21,9.21 29.37,9.37 R6.2 | U2.47 14.58,36.86 15.4,36.04 17.62,36.04 18.57,35.08 18.57,31.75 27.3,23.02 27.3,20.64 27.3,20.16 27.3,9.53 28.42,8.41 29.21,8.41
MISO  (via drill 0.38)
  Top 0.254: U1.16 19.43,55.82 20.16,55.09 20.16,52.23 21.63,50.76 23.36,50.76 23.95,50.16 v26.83,50.16
  Bottom 0.254: v26.83,50.16 36.2,50.16 J6.2
MOSI  (via drill 0.38)
  Top 0.254: U1.15 18.8,55.02 19.37,54.45 19.37,52.07 21.11,50.32 23.18,50.32 v25.4,48.1
  Bottom 0.254: v25.4,48.1 25.56,48.1 26.04,47.62 36.2,47.62 J6.3
N$2
  Top 0.203: R27.2 18.03,44.07 18.16,44.2 19.94,44.2 20.07,44.07 20.07,43.4 C15.1
N$3
  Top 0.203: R6.1 32.7,9.37 33.02,9.68 33.02,14.13 32.7,14.45 31.81,14.45 C9.1
N$6
  Top 0.203: C11.1 32.86,5.71 33.02,5.87 33.02,7.46 32.86,7.62 R10.1
N$7
  Top 0.203: U2.45 15.58,39.16 14.35,40.39 C7.1
N$8
  Top 0.203: U1.7 13.65,46.35 14.76,45.24 15.66,45.24 15.75,45.16
N$15  (via drill 0.38)
  Top 0.203: R2.2 v20.32,22.38 | v12.86,7.46 12.86,5.92 J2.RSV1
  Bottom 0.203: v20.32,22.38 20.32,17.46 12.86,10 v12.86,7.46
N$16
  Top 0.203: U1.8 14.45,47.78 14.61,47.62 15.68,47.62 15.75,47.55
N$17
  Top 0.203: C10.1 18.57,9.21 18.26,9.53 18.26,10.79 18.57,11.11 R7.1
N$19
  Top 0.203: J2.RSV2 5.05,12.25 3.02,14.29 3.02,21.43 4.13,22.54 4.76,22.54 5.08,22.23 R3.2
N$20
  Top 0.203: R8.1 18.57,12.7 18.26,13.02 18.26,14.29 18.57,14.61 C12.1
N$31
  Top 0.203: U1.25 4.5,55.82 4.32,56.01 4.32,58.29 4.7,58.67 D3.A
N$34
  Top 0.203: D2.C 9.41,29.72 R18.2
N$35
  Top 0.203: U2.10 11.24,32.06 10.41,31.24 D2.A
N$36
  Top 0.203: D3.C 7.24,57.28 R26.2
N$39
  Top 0.254: U1.20 12.05,59.7 10.16,61.59 C16.2
N$42
  Top 0.254: R17.1 31.96,47.33 D1.A
PWRBTN  (via drill 0.38)
  Top 0.203: 19.58,38.63 U2.37 19.58,40.02 v19.94,40.39
  Top 0.254: U1.11 16.9,51.82 17.27,52.2 v17.27,52.32
  Bottom 0.203: v17.27,52.32 20.32,49.28 20.32,47.12 21.34,46.1 21.34,44.58 19.94,43.18 v19.94,40.39
R_AC
  Top 0.203: C10.2 22.54,9.21 22.86,8.89 22.86,7.3 | 22.86,7.3 22.86,6.19 | 22.86,6.19 22.86,4.89 J1.RING | R4.2 22.86,7.3 | J3.1 36.83,12.38 34.45,10 34.45,5.56 32.86,3.97 28.26,3.97 26.04,6.19 22.86,6.19
RAW  (via drill 0.38)
  Top 0.203: U2.33 22.84,35.06 23.81,36.04 23.81,39.85 24.45,40.48 24.45,45.24 v22.38,47.31
  Top 0.254: J4.P$4 17.78,59.85 18.57,59.05 34.92,59.05 J9.2 35.56,55.88 33.66,55.88 33.02,56.52 27.81,56.52 | U3.1 27.78,56.48 27.81,56.52 | 25.91,56.52 27.81,56.52 | U3.3 25.88,56.49 25.91,56.52 | C3.1 22.45,56.23 22.73,56.52 v24.13,56.52 25.91,56.52
  Bottom 0.254: v22.38,47.31 22.38,54.9 24,56.52 v24.13,56.52
RIGHT  (via drill 0.38)
  Top 0.203: R7.2 22.23,11.11 22.38,11.27 22.38,11.91 | 22.38,11.91 22.38,12.54 22.23,12.7 R8.2 | U2.40 18.08,36.69 19.05,35.72 19.05,31.91 28.1,22.86 28.1,19.53 v28.42,19.21 | v23.34,12.06 22.54,12.06 22.38,11.91
  Bottom 0.203: v28.42,19.21 28.42,17.14 v23.34,12.06
RST  (via drill 0.38)
  Top 0.203: U1.29 6.11,52.62 5.71,52.23 5.71,46.99 4.29,45.56 v4.29,43.5 4.29,41.15 4.32,41.12 | C8.2 R9.1 | v20.16,57.63 20.32,57.78 30,57.78 v30.16,57.63 | 4.32,41.12 2.06,41.12 J12.1 | S1.3 4.32,41.12
  Top 0.254: R9.1 31.59,60.33 v32.23,60.96
  Bottom 0.203: 15.56,52.86 15.56,53.02 v20.16,57.63 | v30.16,57.63 30.48,57.63 32.23,59.37 v32.23,60.96 | 13.49,50.8 11.43,48.74 9.53,48.74 8.89,48.1
  Bottom 0.254: 15.56,52.86 13.49,50.8 | 8.89,48.1 v4.29,43.5
RXI  (via drill 0.38)
  Top 0.203: U1.30 8.17,51.82 v9.21,52.86
  Bottom 0.254: v9.21,52.86 12.06,52.86 20,60.8 20,61.91 J4.P$3
SCK  (via drill 0.38)
  Top 0.203: U1.17 14.45,58.11 14.76,58.42 32.86,58.42 v33.02,58.26
  Top 0.254: R17.2 29.05,48.9 v28.73,49.21
  Bottom 0.254: 33.02,51.75 26.51,51.75 25.4,50.64 25.4,49.53 25.72,49.21 v28.73,49.21 | 33.02,51.75 36.51,51.75 J6.1 | v33.02,58.26 33.02,51.75
SCL
  Top 0.203: U1.28 5.48,53.42 5.08,53.02 5.08,48.26 J7.1
SCLK  (via drill 0.38)
  Top 0.203: U2.23 19.08,28.86 19.68,28.26 19.68,25.72 20,25.4 21.43,25.4 v22.38,24.45 | U4.6 34.11,27.53 v34.36,27.77
  Bottom 0.203: v22.38,24.45 31.43,24.45 33.02,26.04 33.02,26.43 v34.36,27.77
SDA
  Top 0.203: U1.27 5.33,54.22 4.45,53.34 4.45,50.16 J7.2
SDCD  (via drill 0.38)
  Top 0.203: U2.21 18.08,28.59 18.57,28.1 18.57,24.13 v19.37,23.34 | v10.16,22.38 R24.1 | J2.CD1 7.38,16.11 v7.46,16.19
  Bottom 0.203: v7.46,16.19 7.46,19.68 v10.16,22.38 10.16,27.3 10.48,27.62 17.62,27.62 18.1,27.15 18.1,24.61 v19.37,23.34
SDCK  (via drill 0.38)
  Top 0.203: U2.14 14.58,24.58 12.86,22.86 v12.7,22.86 R20.1 | J2.SCLK 8.35,14.86 v8.57,15.08
  Bottom 0.203: v8.57,15.08 8.57,15.24 8.89,15.24 12.7,19.05 v12.7,22.86
SDDI  (via drill 0.38)
  Top 0.203: U2.16 15.58,23.34 v15.58,22.7 15.58,22.56 15.24,22.23 R19.1 | J2.DI 10.55,13.09 v11.27,13.81
  Bottom 0.203: v11.27,13.81 11.27,14.76 15.24,18.73 15.24,22.36 v15.58,22.7
SDDO
  Top 0.203: U2.13 14.08,28.84 8.18,22.94 | 8.18,22.94 7.62,22.38 R21.1 | J2.DO 6.15,13.38 4.13,15.4 4.13,17.46 4.45,17.78 5.56,17.78 6.51,18.73 6.51,22.86 6.99,23.34 7.78,23.34 8.18,22.94
SDXCS  (via drill 0.38)
  Top 0.203: U2.20 17.58,28.46 18.1,27.94 v18.1,22.7 18.1,22.54 17.78,22.23 R13.1 | J2.CS 11.65,11.97 v13.81,14.13
  Bottom 0.203: v13.81,14.13 13.81,15.56 17.78,19.53 17.78,22.38 v18.1,22.7
SI  (via drill 0.38)
  Top 0.203: U2.24 19.58,29 20,28.57 20.16,28.57 v22.7,26.04 | U4.2 24.35,28.8 v24.13,28.57
  Bottom 0.203: 22.86,26.19 v22.7,26.04 23.81,27.15 23.81,28.26 v24.13,28.57
SO
  Top 0.203: U2.25 22.01,31.06 23.63,29.44 29.03,29.44 32.16,26.31 32.16,26.26 U4.5
TXO  (via drill 0.38)
  Top 0.254: U1.31 9.11,51.02 v9.68,51.59
  Bottom 0.254: v9.68,51.59 12.38,51.59 21.43,60.64 21.43,60.8 J4.P$2
USBN  (via drill 0.38)
  Top 0.203: U2.36 21.8,36.56 22.23,36.99 22.23,37.31 21.91,37.62 v20.8,37.62 | J10.2 35.88,30.16 35.88,30.96 34.77,32.07 34.77,35.24 v35.72,36.2
  Bottom 0.203: v20.8,37.62 32.7,37.62 34.13,36.2 v35.72,36.2
USBP  (via drill 0.38)
  Top 0.203: U2.35 22.41,36.06 v22.7,36.35 | v30.8,25.56 31.59,25.56 31.91,25.24 v33.66,25.24
  Bottom 0.203: v22.7,36.35 25.88,36.35 26.67,35.56 26.67,29.69 24.61,27.62 24.61,27.3 26.67,25.24 30.48,25.24 v30.8,25.56 | v33.66,25.24 35.4,25.24 J10.1
VCC  (via drill 0.38)
  Top 0.203: R3.1 4.03,19.47 v3.81,19.68 | v9.53,3.02 9.53,5.54 J2.VCC | 11.27,49.85 v11.27,47.15 | 29.05,46.67 v29.21,46.51 | v18.57,60.33 19.37,59.53 26.51,59.53 27.46,60.48 v27.46,60.64 | v17.46,59.21 14.13,59.21 13.65,58.74 U1.18 | v22.38,19.53 20.32,19.53 R2.1 | v31.27,22.86 30.8,23.34 30.8,24.61 30,25.4 30,25.72 v30.8,26.51 | 26.1,27.53 v26.04,27.46 | U4.7 32,28.8 31.75,29.05 31.75,29.84 31.97,30.07 U4.8 34.04,30.07 v34.13,30.16
  Top 0.254: U1.18 13.65,52.23 12.46,51.04 | 12.46,51.04 11.27,49.85 11.27,48.75 U1.4 | U1.6 12.85,50.65 12.46,51.04 | R9.2 27.78,60.33 v27.46,60.64 | U3.5 27.78,50.8 | v29.21,46.51 27.78,47.95 27.78,50.8 | v28.89,54.13 28.89,52.23 | C14.1 28.89,52.23 | 28.89,52.23 28.89,51.12 28.57,50.8 27.78,50.8 | 15.88,31.5 v15.88,31.37 16.08,31.17 U2.17 | v12.57,28.32 12.57,27.94 9.14,24.51 v8.13,24.51 | U4.3 26.04,27.53 v26.04,27.46
  Bottom 0.203: v11.27,47.15 10,47.15 4.76,41.91 3.65,41.91 3.02,42.55 3.02,47.78 J7.3 | v29.21,46.51 29.21,45.4 36.83,37.78 J5.2 34.09,34.29 | v27.46,60.64 27.46,57.94 28.89,56.52 v28.89,54.13 | v3.81,19.68 4.03,19.47 R3.1 5.87,18.68 5.87,16.03 9.53,12.38 v9.53,3.02 10.48,3.02 22.38,14.92 v22.38,19.53 26.04,23.18 29.84,23.18 30.16,23.5 30.64,23.5 v31.27,22.86 | 30.8,27.3 v30.8,26.51 | 30.8,27.3 29.37,27.3 29.05,26.99 26.51,26.99 v26.04,27.46 | v18.57,60.33 v17.46,59.21 | 30.8,27.3 30.8,33.02 32.07,34.29 34.09,34.29 | v34.13,30.16 34.13,34.25 34.09,34.29
  Bottom 0.254: v15.88,31.37 12.83,28.32 v12.57,28.32 | v8.13,24.51 8.13,22.61 5.08,19.56 R3.1
VS_RX
  Top 0.203: U2.27 22.7,32.06 23.34,31.43 28.73,31.43 29.21,30.96 34.61,30.96 35.08,30.48 35.08,25.88 J11.2 31.81,24.13 R16.1 31.43,24.19
VS_TX  (via drill 0.38)
  Top 0.203: U2.26 22.41,31.56 23.34,30.64 24.13,30.64 24.29,30.8 28.42,30.8 v28.57,30.64 | v28.73,28.42 28.73,22.86 29.84,21.75 36.67,21.75 J11.1
  Bottom 0.203: v28.57,30.64 28.57,28.57 v28.73,28.42
XCS  (via drill 0.38)
  Top 0.203: U2.22 18.58,28.73 19.21,28.1 19.21,24.92 19.61,24.53 20.72,24.53 v20.8,24.45 20.95,24.29 20.95,23.18 21.27,22.86 R25.1 | U4.1 27.27,30 25.2,30 v25.08,30.12
  Bottom 0.203: v25.08,30.12 24.96,30 23.81,30 21.91,28.1 19.53,28.1 19.21,27.78 19.21,24.92 19.68,24.45 v20.8,24.45
XRST
  Top 0.203: U2.1 8.2,36.56 5.33,39.43 C13.1 | R23.1 1.62,37.53 2.41,38.32 2.41,38.58 C13.1 | 3.33,39.5 C13.1
XTAL0
  Top 0.203: U2.29 23.54,33.06 25.4,34.92 26.45,34.92 R1.1 27.36,34.98 28.1,35.72 28.1,40.48 29.37,41.75 33.18,41.75 33.66,41.27 33.66,40.86 | 33.66,40.86 33.66,39.04 Y1.1 | C2.2 33.59,40.8 33.66,40.86
XTAL1
  Top 0.203: U2.28 23.16,32.56 23.65,32.07 26.51,32.07 | 26.51,32.07 28.57,32.07 | 28.57,32.07 29.79,32.07 C1.2 | R1.2 26.51,32.07 | Y1.3 30.06,34.66 28.57,33.18 28.57,32.07

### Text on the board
Bottom: v10
tPlace: RDY | A0 | VIN | A1 | GND | PAPA / SOUNDIE | GND | SCK / D13 | 3.3V | MISO / D12 | SDA | RST | MOSI / D11 | SCL | D10 | RST | D9 | 3.3V | VLSI RDY | GND | UN | UP | RX | TX | L | R
bPlace: A0 | VIN | A1 | GND | GND | SCK / D13 | 3.3V | MISO / D12 | SDA | MOSI / D11 | SCL | PAPA / SOUNDIE | D10 | RST | D9 | Audio Player | 3.3V | GND | USBN | USBP | VS_RX | VS_TX | LEFT_AC | RIGHT_AC
Measures: All Units Inches
tDocu: Mary West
